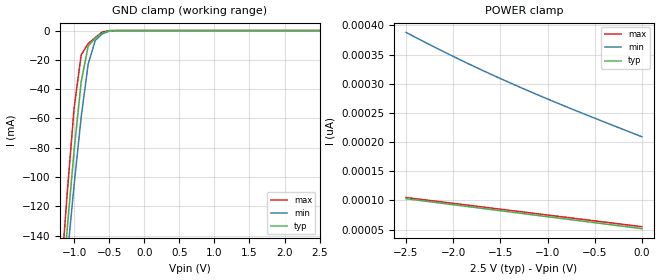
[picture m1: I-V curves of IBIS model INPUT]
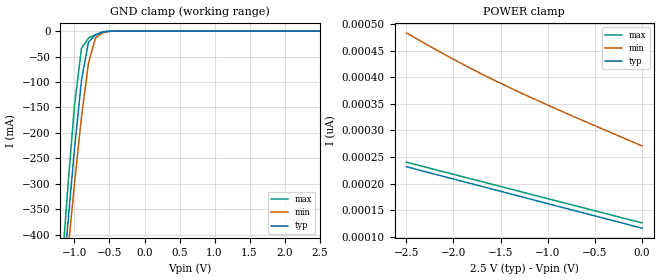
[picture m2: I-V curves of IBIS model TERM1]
|   PERICOM SEMICONDUCTOR CORP
|   IBIS Model of PI3C3306
|   Product Family: 3C
|   MSOP (U) Package
[IBIS Ver] 3.2
[Comment char] |_char
[File Name] pi3c3306_u_25v.ibs
[File Rev] 1.0
[Source] File originated at Pericom Semiconductor Corp.
[Date] 12/25/17
[Disclaimer] (C) Copyright PERICOM Semiconductor Corporation
   All rights reserved
  Pericom Semiconductor Corporation hereby grants the user of
  this IBIS model a non-exclusive, nontransferable license to
  use this IBIS model under the following terms.
  This IBIS model is provided on an "AS IS" basis and Pericom
  makes absolutely no warranty with respect to the information
  contained herein. PERICOM DISCLAIMS AND CUSTOMER WAIVES ALL
  WARRANTIES, EXPRESSED OR IMPLIED, INCLUDING WARRANTIES OF
  MERCHANTABILITY OR FITNESS FOR A PARTICULAR PURPOSE. The
  entire risk as to quality and performance is with the customer.
  Accordingly, in no event shall the company be liable for any
  damages, whether in contract or tort, including any lost
  profits or other incidental, consequential, exemplary, or
  punitive damages arising out of the use or application of the
  IBIS model provided in this package. Further, Pericom reserves
  the right to make changes without notice to any product herein
  to improve reliability, function, or design. Pericom does not
  convey any license under patent rights or any other intellectual
  property rights, including those of third parties.
  The user is granted this license only to use the IBIS model
  and is not granted rights to sell, load, rent, lease or license
  the IBIS model in whole or in part, or in modified form to anyone
  other than user. User may modify the IBIS model to suit its specific
  application but rights to derivative works and such modifications
  shall belong to Pericom.
  Pericom is not obligated to provide maintenance or support
  for the licensed IBIS model.
  Contact Pericom at ATTN: APPLICATION ENGINEERING / IBIS MODELS
  2380 Bering Drive, San Jose, CA 95131
[Component] PI3C3306
[Manufacturer] Pericom Semiconductor Corp.
[Package]
| variable   typ   min   max
R_pkg   0.04200   0.03995   0.04405
L_pkg   2.30669n   2.21200n   2.40138n
C_pkg   0.21108p   0.20715p   0.21500p
[Pin] signal_name  model_name   R_pin   L_pin   C_pin
1   _BE1   INPUT   0.04405   2.40138n   0.21500p
2   A1   TERM1   0.03995   2.21200n   0.20715p
3   B1   TERM2   0.03995   2.21200n   0.20715p
4   GND   GND   0.04405   2.40138n   0.21500p
5   A2   TERM1   0.04405   2.40138n   0.21500p
6   B2   TERM2   0.03995   2.21200n   0.20715p
7   _BE2   INPUT   0.03995   2.21200n   0.20715p
8   VCC   POWER   0.04405   2.40138n   0.21500p
[Series Switch Groups]
On 1 /
Off 2 /
[Series Pin Mapping]   pin_2   model_name  function_table_group
2   3   SWITCH1   1
5   6   SWITCH1   2
|   Model SWITCH1
[Model] SWITCH1
Model_type Series_switch
| variable   typ   min   max
C_comp   10.000pF   9.800pF   10.200pF
[Voltage Range]   2.5000V   2.2500V   2.7500V
[GND Clamp Reference]   0.0000V   0.0000V   0.0000V
[POWER Clamp Reference]   2.5000V   2.2500V   2.7500V
[Temperature Range]   25   85   -40
[On]
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[OFF]
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| Models and submodels in the file (4): INPUT (Input), SWITCH1 (Series_switch), TERM1 (Terminator), TERM2 (Terminator)
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|   Model INPUT
[Model] INPUT
Model_type Input
Vinl = 750mV
Vinh = 1.80V
| variable   typ   min   max
C_comp   3.500pF   3.400pF   3.600pF
[Voltage Range]   2.5000V   2.2500V   2.7500V
[GND Clamp Reference]   0.0000V   0.0000V   0.0000V
[POWER Clamp Reference]   2.5000V   2.2500V   2.7500V
[Temperature Range]   25   85   -40
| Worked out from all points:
|   GND clamp passes 1 mA (typ) near -0.56 V on its own axis
[GND Clamp]
| Voltage   I(typ)   I(min)   I(max)
-2.5V     -998.2mA   -927.2mA   -1.099A
-1.2V     -193.5mA   -207.1mA   -176.6mA
-1.1V     -135.8mA   -155mA     -111.4mA
-1V       -81.33mA   -105mA     -52.61mA
-900mV    -34.92mA   -59.01mA   -16.58mA
-800mV    -10.56mA   -22.8mA    -8.882mA
-700mV    -5.104mA   -6.74mA    -4.717mA
-600mV    -1.611mA   -2.212mA   -981.9uA
-500mV    -145.9uA   -381.4uA   -24.42uA
-400mV    -4.329uA   -29.72uA   -133.6nA
2.5V      51.65pA    224.9pA    50pA
[POWER Clamp]   |Note: Vtable = Vcc - Voutput
| Voltage   I(typ)   I(min)   I(max)
-2.5V     103.1pA    388pA      105pA
-2V       92.73pA    346.8pA    95pA
-1.7V     86.54pA    323.7pA    89pA
-1.4V     80.36pA    301.7pA    83pA
-800mV    68.04pA    260.5pA    71pA
0V        51.65pA    209.1pA    55pA
|   Model TERM1
[Model] TERM1
Model_type Terminator
| variable   typ   min   max
C_comp   5.000pF   4.900pF   5.100pF
[Voltage Range]   2.5000V   2.2500V   2.7500V
[GND Clamp Reference]   0.0000V   0.0000V   0.0000V
[POWER Clamp Reference]   2.5000V   2.2500V   2.7500V
[Temperature Range]   25   85   -40
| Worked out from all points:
|   GND clamp passes 1 mA (typ) near -0.54 V on its own axis
[GND Clamp]
| Voltage   I(typ)   I(min)   I(max)
-2.5V     -2.832A    -2.628A    -3.121A
-1.2V     -551.9mA   -590.4mA   -503.2mA
-1.1V     -387.8mA   -442.8mA   -316.8mA
-1V       -232.2mA   -300.6mA   -146.4mA
-900mV    -97.23mA   -169.1mA   -34.28mA
-800mV    -21.65mA   -63.17mA   -13.78mA
-700mV    -7.82mA    -13.64mA   -7.205mA
-600mV    -2.298mA   -3.355mA   -1.407mA
-500mV    -202.1uA   -564.7uA   -32.57uA
2.5V      116pA      289.9pA    114.4pA
[POWER Clamp]   |Note: Vtable = Vcc - Voutput
| Voltage   I(typ)   I(min)   I(max)
-2.5V     231.7pA    483.7pA    240.3pA
-2V       208.5pA    434.1pA    217.4pA
-1.5V     185.4pA    388.8pA    194.5pA
-900mV    157.6pA    339.9pA    167.1pA
0V        116pA      271pA      125.9pA
